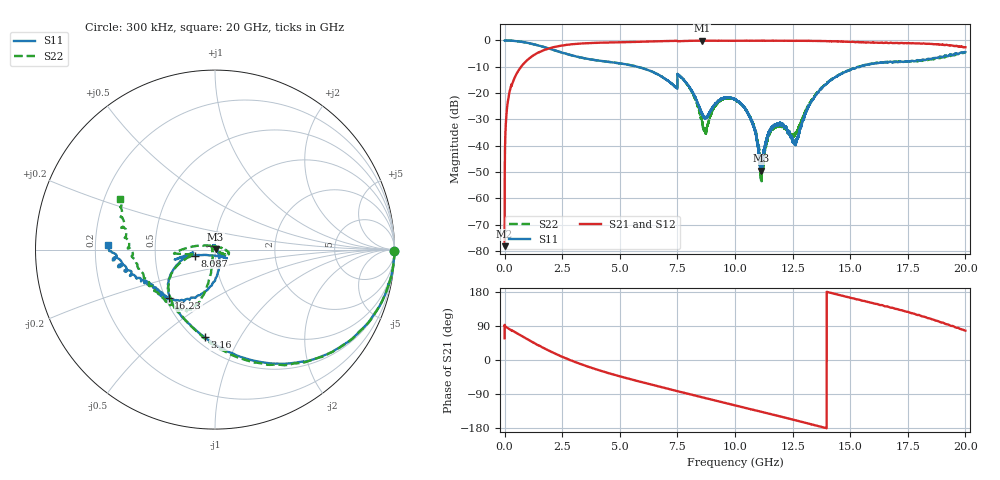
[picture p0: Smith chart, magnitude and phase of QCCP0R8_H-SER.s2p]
!{QCCP0R8}
!Johanson Technology Inc.
!www.johansontechnology.com
!Test Board Conditions:
!Substrate Type  RO4350B
!Substrate Thickness  20 mil
!Substrate Dk  3.66
!TL Type: GCPW
!TL Trace Width  36 mil
!TL Gap  12 mil
!Electrode orientation  Horizontal
!DUT TOPOLOGY	SERIES
!Mounting Pad LxW  26x36 mil
! Created Sat Jan  9 18:24:35 2021
# hz S ma R 50
! 2 Port Network Data from SP1.SP block
! freq  magS11  angS11  magS21  angS21  magS12  angS12  magS22  angS22
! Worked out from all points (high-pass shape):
!   20001 points, 300 kHz to 20 GHz, reference 50 ohm
!   highest |S21| = -0.07 dB at 8.57 GHz (marker M1); lowest = -78.1 dB at 300 kHz (marker M2)
!   |S21| within 3 dB of the highest: 1.91 GHz to end of sweep
!   lowest |S11| = -49.5 dB at 11.13 GHz (marker M3), VSWR 1.01, Z = 50.3 + j0.111 ohm
!   |S11| at or under -10 dB: 5.761714 GHz to 5.762589 GHz (874.9 kHz wide, 0.0152 % of centre); 5.765 GHz to 15.43 GHz (9.666 GHz wide, 91.2 % of centre)
!   |S22| runs from -53.7 to 0.0 dB; largest |S21 - S12| = 0.02
!   S11 on the Smith chart (normalised r, x): 300 kHz: open; 3.16 GHz: 0.56, -0.72; 8.087 GHz: 0.80, -0.05; 16.23 GHz: 0.52, -0.33; 20 GHz: 0.25, +0.02
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300000  0.9957 -0.3  0.0001242 57.3  0.0001577 126.6  0.9972 -0.4
1.303e8  0.9976 -5.1  0.06462 84.6  0.0647 84.7  0.9976 -5.0
4.893e8  0.9739 -17.3  0.2196 72.4  0.2195 72.3  0.9734 -17.3
1.5713e9  0.78 -53.6  0.6162 35.6  0.617 35.7  0.7782 -54.4
3.1603e9  0.4904 -96.8  0.866 -7.5  0.8657 -7.5  0.4912 -98.0
3.3343e9  0.472 -100.9  0.876 -11.5  0.8754 -11.5  0.472 -101.9
6.6673e9  0.2257 -158.4  0.9663 -69.3  0.9669 -69.3  0.2238 -157.6
8.0873e9  0.1175 -163.5  0.9837 -91.1  0.9843 -91.0  0.1133 170.3
8.5703e9  0.04116 -129.6  0.9921 -98.4  0.9903 -98.3  0.02882 130.4
8.7153e9  0.03392 -96.5  0.9887 -100.5  0.9902 -100.5  0.01812 74.1
9.2403e9  0.06849 -40.6  0.9873 -108.4  0.9866 -108.3  0.0639 -5.2
1.00003e10  0.07471 -38.7  0.9859 -119.7  0.9874 -119.7  0.07488 -21.7
1.07313e10  0.02834 -38.7  0.99 -130.6  0.989 -130.7  0.02943 -33.1
1.11253e10  0.00336 19.1  0.9868 -136.5  0.9889 -136.5  0.00285 11.4
1.15693e10  0.02171 111.8  0.9867 -143.0  0.9857 -143.0  0.02004 129.8
1.20253e10  0.0247 102.3  0.9863 -149.9  0.9869 -149.9  0.02259 135.8
1.26153e10  0.01068 20.8  0.9849 -159.0  0.9858 -158.9  0.01659 -157.1
1.33343e10  0.07133 -69.2  0.9801 -170.0  0.9794 -170.1  0.07428 -100.8
1.45513e10  0.2254 -100.2  0.9557 171.1  0.9559 171.2  0.2263 -103.2
1.62313e10  0.374 -133.6  0.9011 146.3  0.9042 146.2  0.376 -115.8
1.66673e10  0.3852 -139.8  0.8906 140.2  0.8963 139.7  0.3885 -121.2
2e10  0.5974 177.1  0.7439 77.5  0.7371 77.6  0.5997 151.9
